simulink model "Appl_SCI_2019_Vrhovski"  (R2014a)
settings: Solver=ode45  StartTime=0.0  StopTime=1000  MaxStep=0.01  RelTol=1e-3
undefined symbols (not defined in the file): deg, H, kg, m, M, mm, N, rad, s, X, Y, Z
libraries: sm_lib x389, nesl_utility x69, simulink x7
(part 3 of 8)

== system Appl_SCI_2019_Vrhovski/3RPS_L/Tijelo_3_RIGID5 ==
  ReferenceFrame : sm_lib/Frames and Transforms/Reference Frame  BlockFunction=simmechanics.library.frames_transforms.reference_frame
  Solid : sm_lib/Body Elements/Solid  InertiaType=Custom  Mass=3.25  MassUnits=kg  CenterOfMass=[0 67.696607712724699 0]  CenterOfMassUnits=mm  MomentsOfInertia=[7450 490 7450]  MomentsOfInertiaUnits=kg*mm^2  ProductsOfInertia=[0 0 0]  ProductsOfInertiaUnits=kg*mm^2  DensityBased=on  Density=1000  DensityUnits=kg/(m^3)  GraphicType=FromGeometry  MarkerShape=Sphere  MarkerSize=10  MarkerSizeUnits=m  GraphicVisPropType=SimpleVisualProperties  GraphicDiffuseColor=[0.4 0.4 0.4]  GraphicSpecularColor=[0.5 0.5 0.5 1.0]  GraphicAmbientColor=[0.15 0.15 0.15 1.0]  GraphicEmissiveColor=[0.0 0.0 0.0 1.0]  GraphicShininess=75  GraphicOpacity=1  GeometryShape=Cylinder  RectangleSize=[1 1]  RectangleSizeUnits=m  BrickDimensions=[1 1 1]  BrickDimensionUnits=m  CylinderRadius=15  CylinderRadiusUnits=mm  CylinderLength=280  CylinderLengthUnits=mm  SphereRadius=1  SphereRadiusUnits=m  EllipsoidRadii=[1 1 1]  EllipsoidRadiiUnits=m  ExtrusionCrossSection=[1 1; -1 1; -1 -1; 1 -1]  ExtrusionCrossSectionUnits=m  ExtrusionLength=1  ExtrusionLengthUnits=m  PolygonNumSides=3  PolygonOuterRadius=1  PolygonOuterRadiusUnits=m  ExtGeomFileType=STL  ExtGeomFileName=Tijelo_Default_sldprt.STL  ExtGeomFileUnits=mm  RevolutionCrossSection=[1 1; 1 -1; 2 -1; 2 1]  RevolutionCrossSectionUnits=m  RevolutionExtent=Full  RevolutionAngle=180  RevolutionAngleUnits=deg  BlockFunction=simmechanics.library.body_elements.solid
  Transform : sm_lib/Frames and Transforms/Rigid Transform  TranslationMethod=StandardAxis  TranslationLengthUnit=mm  TranslationStandardAxis=-Z  TranslationStandardOffset=13.29  TranslationCartesianOffset=[0 10 0]  TranslationROffset=0  TranslationROffsetUnits=m  TranslationZOffset=0  TranslationZOffsetUnits=m  TranslationThetaOffset=0  TranslationThetaOffsetUnits=deg  RotationMethod=None  RotationAngleUnits=rad  RotationStandardAxis=+Z  RotationAngle=2.0943951023931953  RotationArbitraryAxis=[-0.57735026918962584 -0.57735026918962584 -0.57735026918962584]  FollAlignAxisA=+X  BaseAlignAxisA=+Y  FollAlignAxisB=+Y  BaseAlignAxisB=+Z  BlockFunction=simmechanics.library.frames_transforms.rigid_transform
  Transform1 : sm_lib/Frames and Transforms/Rigid Transform  TranslationMethod=None  TranslationLengthUnit=mm  TranslationStandardAxis=+Z  TranslationStandardOffset=0  TranslationCartesianOffset=[0 100 0]  TranslationROffset=0  TranslationROffsetUnits=m  TranslationZOffset=0  TranslationZOffsetUnits=m  TranslationThetaOffset=0  TranslationThetaOffsetUnits=deg  RotationMethod=None  RotationAngleUnits=rad  RotationStandardAxis=+Z  RotationAngle=3.1415926535897905  RotationArbitraryAxis=[1 -1.4003819427637228e-30 -9.8290662577982061e-16]  FollAlignAxisA=+X  BaseAlignAxisA=+Y  FollAlignAxisB=+Y  BaseAlignAxisB=+Z  BlockFunction=simmechanics.library.frames_transforms.rigid_transform
  F1 : PMIOPort  Port=1  Side=Left
  F : PMIOPort  Port=2  Side=Right
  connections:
  Transform1/RConn1 -- F1/RConn1
  Transform/RConn1 -- F/RConn1
  Transform1/LConn1 -- Solid/RConn1 -- ReferenceFrame/RConn1 -- Transform/LConn1

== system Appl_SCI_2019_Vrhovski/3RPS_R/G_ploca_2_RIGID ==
  ReferenceFrame : sm_lib/Frames and Transforms/Reference Frame  BlockFunction=simmechanics.library.frames_transforms.reference_frame
  Solid : sm_lib/Body Elements/Solid  InertiaType=Custom  Mass=5  MassUnits=kg  CenterOfMass=[-1.0925911726464245e-05 0 -4.4436244658035022]  CenterOfMassUnits=mm  MomentsOfInertia=[45540 79860 45540]  MomentsOfInertiaUnits=kg*mm^2  ProductsOfInertia=[0 -0.00010369999054466602 0]  ProductsOfInertiaUnits=kg*mm^2  DensityBased=on  Density=1000  DensityUnits=kg/(m^3)  GraphicType=FromGeometry  MarkerShape=Sphere  MarkerSize=10  MarkerSizeUnits=m  GraphicVisPropType=SimpleVisualProperties  GraphicDiffuseColor=[0.4 0.4 0.4]  GraphicSpecularColor=[0.5 0.5 0.5 1.0]  GraphicAmbientColor=[0.15 0.15 0.15 1.0]  GraphicEmissiveColor=[0.0 0.0 0.0 1.0]  GraphicShininess=75  GraphicOpacity=1  GeometryShape=Brick  RectangleSize=[1 1]  RectangleSizeUnits=m  BrickDimensions=[240 210 20]  BrickDimensionUnits=mm  CylinderRadius=120  CylinderRadiusUnits=mm  CylinderLength=20  CylinderLengthUnits=mm  SphereRadius=1  SphereRadiusUnits=m  EllipsoidRadii=[1 1 1]  EllipsoidRadiiUnits=m  ExtrusionCrossSection=[1 1; -1 1; -1 -1; 1 -1]  ExtrusionCrossSectionUnits=m  ExtrusionLength=1  ExtrusionLengthUnits=m  PolygonNumSides=3  PolygonOuterRadius=1  PolygonOuterRadiusUnits=m  ExtGeomFileType=STL  ExtGeomFileName=G_ploca_Default_sldprt.STL  ExtGeomFileUnits=mm  RevolutionCrossSection=[1 1; 1 -1; 2 -1; 2 1]  RevolutionCrossSectionUnits=m  RevolutionExtent=Full  RevolutionAngle=180  RevolutionAngleUnits=deg  BlockFunction=simmechanics.library.body_elements.solid
  Transform : sm_lib/Frames and Transforms/Rigid Transform  TranslationMethod=Cartesian  TranslationLengthUnit=mm  TranslationStandardAxis=+Z  TranslationStandardOffset=0  TranslationCartesianOffset="[-50.0000   -86.6025         -10]"  TranslationROffset=0  TranslationROffsetUnits=m  TranslationZOffset=0  TranslationZOffsetUnits=m  TranslationThetaOffset=0  TranslationThetaOffsetUnits=deg  RotationMethod=ArbitraryAxis  RotationAngleUnits=rad  RotationStandardAxis=+Z  RotationAngle=0  RotationArbitraryAxis=[0 0 0]  FollAlignAxisA=+X  BaseAlignAxisA=+Y  FollAlignAxisB=+Y  BaseAlignAxisB=+Z  BlockFunction=simmechanics.library.frames_transforms.rigid_transform
  Transform1 : sm_lib/Frames and Transforms/Rigid Transform  TranslationMethod=Cartesian  TranslationLengthUnit=mm  TranslationStandardAxis=+Z  TranslationStandardOffset=0  TranslationCartesianOffset="[-50.0000   86.6025         -10]"  TranslationROffset=0  TranslationROffsetUnits=m  TranslationZOffset=0  TranslationZOffsetUnits=m  TranslationThetaOffset=0  TranslationThetaOffsetUnits=deg  RotationMethod=ArbitraryAxis  RotationAngleUnits=rad  RotationStandardAxis=+Z  RotationAngle=0  RotationArbitraryAxis=[0 0 0]  FollAlignAxisA=+X  BaseAlignAxisA=+Y  FollAlignAxisB=+Y  BaseAlignAxisB=+Z  BlockFunction=simmechanics.library.frames_transforms.rigid_transform
  Transform2 : sm_lib/Frames and Transforms/Rigid Transform  TranslationMethod=Cartesian  TranslationLengthUnit=mm  TranslationStandardAxis=+Z  TranslationStandardOffset=0  TranslationCartesianOffset=[100 0 -10]  TranslationROffset=0  TranslationROffsetUnits=m  TranslationZOffset=0  TranslationZOffsetUnits=m  TranslationThetaOffset=0  TranslationThetaOffsetUnits=deg  RotationMethod=ArbitraryAxis  RotationAngleUnits=rad  RotationStandardAxis=+Z  RotationAngle=0  RotationArbitraryAxis=[0 0 0]  FollAlignAxisA=+X  BaseAlignAxisA=+Y  FollAlignAxisB=+Y  BaseAlignAxisB=+Z  BlockFunction=simmechanics.library.frames_transforms.rigid_transform
  Transform3 : sm_lib/Frames and Transforms/Rigid Transform  TranslationMethod=StandardAxis  TranslationLengthUnit=mm  TranslationStandardAxis=+Z  TranslationStandardOffset=10  TranslationCartesianOffset=[80.000000000002558 4.2632564145606011e-14 -32.999999999999048]  TranslationROffset=0  TranslationROffsetUnits=m  TranslationZOffset=0  TranslationZOffsetUnits=m  TranslationThetaOffset=0  TranslationThetaOffsetUnits=deg  RotationMethod=None  RotationAngleUnits=rad  RotationStandardAxis=+Z  RotationAngle=0  RotationArbitraryAxis=[0 0 0]  FollAlignAxisA=+X  BaseAlignAxisA=+Y  FollAlignAxisB=+Y  BaseAlignAxisB=+Z  BlockFunction=simmechanics.library.frames_transforms.rigid_transform
  F2 : PMIOPort  Port=1  Side=Left
  F1 : PMIOPort  Port=2  Side=Left
  F : PMIOPort  Port=3  Side=Left
  F3 : PMIOPort  Port=4  Side=Right
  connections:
  ReferenceFrame/RConn1 -- Transform/LConn1 -- Transform1/LConn1 -- Transform2/LConn1 -- Transform3/LConn1 -- Solid/RConn1
  Transform/RConn1 -- F/RConn1
  Transform1/RConn1 -- F1/RConn1
  Transform2/RConn1 -- F2/RConn1
  Transform3/RConn1 -- F3/RConn1

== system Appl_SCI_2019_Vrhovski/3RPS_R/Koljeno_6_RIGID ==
  ReferenceFrame : sm_lib/Frames and Transforms/Reference Frame  BlockFunction=simmechanics.library.frames_transforms.reference_frame
  Solid : sm_lib/Body Elements/Solid  InertiaType=Custom  Mass=1.2  MassUnits=kg  CenterOfMass=[0 94.726347166305388 0]  CenterOfMassUnits=mm  MomentsOfInertia=[342 72 342]  MomentsOfInertiaUnits=kg*mm^2  ProductsOfInertia=[0 0 0]  ProductsOfInertiaUnits=kg*mm^2  DensityBased=on  Density=1000  DensityUnits=kg/(m^3)  GraphicType=FromGeometry  MarkerShape=Sphere  MarkerSize=10  MarkerSizeUnits=m  GraphicVisPropType=SimpleVisualProperties  GraphicDiffuseColor=[0.792156862745098 0.81960784313725488 0.93333333333333335]  GraphicSpecularColor=[0.5 0.5 0.5 1.0]  GraphicAmbientColor=[0.15 0.15 0.15 1.0]  GraphicEmissiveColor=[0.0 0.0 0.0 1.0]  GraphicShininess=75  GraphicOpacity=1  GeometryShape=FromFile  RectangleSize=[1 1]  RectangleSizeUnits=m  BrickDimensions=[1 1 1]  BrickDimensionUnits=m  CylinderRadius=1  CylinderRadiusUnits=m  CylinderLength=1  CylinderLengthUnits=m  SphereRadius=1  SphereRadiusUnits=m  EllipsoidRadii=[1 1 1]  EllipsoidRadiiUnits=m  ExtrusionCrossSection=[1 1; -1 1; -1 -1; 1 -1]  ExtrusionCrossSectionUnits=m  ExtrusionLength=1  ExtrusionLengthUnits=m  PolygonNumSides=3  PolygonOuterRadius=1  PolygonOuterRadiusUnits=m  ExtGeomFileType=STL  ExtGeomFileName=E:\Fer 2\Doktorski studij\Doktorat\LLD\matlab\LLD 3RPS\PS_limb.STL  ExtGeomFileUnits=mm  RevolutionCrossSection=[1 1; 1 -1; 2 -1; 2 1]  RevolutionCrossSectionUnits=m  RevolutionExtent=Full  RevolutionAngle=180  RevolutionAngleUnits=deg  BlockFunction=simmechanics.library.body_elements.solid
  Transform : sm_lib/Frames and Transforms/Rigid Transform  TranslationMethod=Cartesian  TranslationLengthUnit=mm  TranslationStandardAxis=+Z  TranslationStandardOffset=0  TranslationCartesianOffset=[2.9560869854197764e-13 -4.9068237247312261e-13 -4.0348858674063459e-14]  TranslationROffset=0  TranslationROffsetUnits=m  TranslationZOffset=0  TranslationZOffsetUnits=m  TranslationThetaOffset=0  TranslationThetaOffsetUnits=deg  RotationMethod=ArbitraryAxis  RotationAngleUnits=rad  RotationStandardAxis=+Z  RotationAngle=2.0943951023931988  RotationArbitraryAxis=[-0.57735026918962673 -0.57735026918962595 -0.57735026918962451]  FollAlignAxisA=+X  BaseAlignAxisA=+Y  FollAlignAxisB=+Y  BaseAlignAxisB=+Z  BlockFunction=simmechanics.library.frames_transforms.rigid_transform
  Transform1 : sm_lib/Frames and Transforms/Rigid Transform  TranslationMethod=Cartesian  TranslationLengthUnit=mm  TranslationStandardAxis=+Z  TranslationStandardOffset=0  TranslationCartesianOffset=[0 162 0]  TranslationROffset=0  TranslationROffsetUnits=m  TranslationZOffset=0  TranslationZOffsetUnits=m  TranslationThetaOffset=0  TranslationThetaOffsetUnits=deg  RotationMethod=ArbitraryAxis  RotationAngleUnits=rad  RotationStandardAxis=+Z  RotationAngle=0  RotationArbitraryAxis=[0 0 0]  FollAlignAxisA=+X  BaseAlignAxisA=+Y  FollAlignAxisB=+Y  BaseAlignAxisB=+Z  BlockFunction=simmechanics.library.frames_transforms.rigid_transform
  F : PMIOPort  Port=1  Side=Left
  F1 : PMIOPort  Port=2  Side=Right
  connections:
  Solid/RConn1 -- ReferenceFrame/RConn1 -- Transform/LConn1 -- Transform1/LConn1
  Transform/RConn1 -- F/RConn1
  Transform1/RConn1 -- F1/RConn1

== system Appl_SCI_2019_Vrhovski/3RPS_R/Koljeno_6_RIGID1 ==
  ReferenceFrame : sm_lib/Frames and Transforms/Reference Frame  BlockFunction=simmechanics.library.frames_transforms.reference_frame
  Solid : sm_lib/Body Elements/Solid  InertiaType=Custom  Mass=1.2  MassUnits=kg  CenterOfMass=[0 94.726347166305388 0]  CenterOfMassUnits=mm  MomentsOfInertia=[342 72 342]  MomentsOfInertiaUnits=kg*mm^2  ProductsOfInertia=[0 0 0]  ProductsOfInertiaUnits=kg*mm^2  DensityBased=on  Density=1000  DensityUnits=kg/(m^3)  GraphicType=FromGeometry  MarkerShape=Sphere  MarkerSize=10  MarkerSizeUnits=m  GraphicVisPropType=SimpleVisualProperties  GraphicDiffuseColor=[0.792156862745098 0.81960784313725488 0.93333333333333335]  GraphicSpecularColor=[0.5 0.5 0.5 1.0]  GraphicAmbientColor=[0.15 0.15 0.15 1.0]  GraphicEmissiveColor=[0.0 0.0 0.0 1.0]  GraphicShininess=75  GraphicOpacity=1  GeometryShape=FromFile  RectangleSize=[1 1]  RectangleSizeUnits=m  BrickDimensions=[1 1 1]  BrickDimensionUnits=m  CylinderRadius=1  CylinderRadiusUnits=m  CylinderLength=1  CylinderLengthUnits=m  SphereRadius=1  SphereRadiusUnits=m  EllipsoidRadii=[1 1 1]  EllipsoidRadiiUnits=m  ExtrusionCrossSection=[1 1; -1 1; -1 -1; 1 -1]  ExtrusionCrossSectionUnits=m  ExtrusionLength=1  ExtrusionLengthUnits=m  PolygonNumSides=3  PolygonOuterRadius=1  PolygonOuterRadiusUnits=m  ExtGeomFileType=STL  ExtGeomFileName=E:\Fer 2\Doktorski studij\Doktorat\LLD\matlab\LLD 3RPS\PS_limb.STL  ExtGeomFileUnits=mm  RevolutionCrossSection=[1 1; 1 -1; 2 -1; 2 1]  RevolutionCrossSectionUnits=m  RevolutionExtent=Full  RevolutionAngle=180  RevolutionAngleUnits=deg  BlockFunction=simmechanics.library.body_elements.solid
  Transform : sm_lib/Frames and Transforms/Rigid Transform  TranslationMethod=Cartesian  TranslationLengthUnit=mm  TranslationStandardAxis=+Z  TranslationStandardOffset=0  TranslationCartesianOffset=[2.9560869854197764e-13 -4.9068237247312261e-13 -4.0348858674063459e-14]  TranslationROffset=0  TranslationROffsetUnits=m  TranslationZOffset=0  TranslationZOffsetUnits=m  TranslationThetaOffset=0  TranslationThetaOffsetUnits=deg  RotationMethod=ArbitraryAxis  RotationAngleUnits=rad  RotationStandardAxis=+Z  RotationAngle=2.0943951023931988  RotationArbitraryAxis=[-0.57735026918962673 -0.57735026918962595 -0.57735026918962451]  FollAlignAxisA=+X  BaseAlignAxisA=+Y  FollAlignAxisB=+Y  BaseAlignAxisB=+Z  BlockFunction=simmechanics.library.frames_transforms.rigid_transform
  Transform1 : sm_lib/Frames and Transforms/Rigid Transform  TranslationMethod=Cartesian  TranslationLengthUnit=mm  TranslationStandardAxis=+Z  TranslationStandardOffset=0  TranslationCartesianOffset=[0 161.99999999999997 0]  TranslationROffset=0  TranslationROffsetUnits=m  TranslationZOffset=0  TranslationZOffsetUnits=m  TranslationThetaOffset=0  TranslationThetaOffsetUnits=deg  RotationMethod=ArbitraryAxis  RotationAngleUnits=rad  RotationStandardAxis=+Z  RotationAngle=0  RotationArbitraryAxis=[0 0 0]  FollAlignAxisA=+X  BaseAlignAxisA=+Y  FollAlignAxisB=+Y  BaseAlignAxisB=+Z  BlockFunction=simmechanics.library.frames_transforms.rigid_transform
  F : PMIOPort  Port=1  Side=Left
  F1 : PMIOPort  Port=2  Side=Right
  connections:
  Transform1/RConn1 -- F1/RConn1
  Transform/RConn1 -- F/RConn1
  Solid/RConn1 -- ReferenceFrame/RConn1 -- Transform1/LConn1 -- Transform/LConn1

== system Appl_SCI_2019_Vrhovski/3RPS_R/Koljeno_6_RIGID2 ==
  ReferenceFrame : sm_lib/Frames and Transforms/Reference Frame  BlockFunction=simmechanics.library.frames_transforms.reference_frame
  Solid : sm_lib/Body Elements/Solid  InertiaType=Custom  Mass=1.2  MassUnits=kg  CenterOfMass=[0 94.726347166305388 0]  CenterOfMassUnits=mm  MomentsOfInertia=[342 72 342]  MomentsOfInertiaUnits=kg*mm^2  ProductsOfInertia=[0 0 0]  ProductsOfInertiaUnits=kg*mm^2  DensityBased=on  Density=1000  DensityUnits=kg/(m^3)  GraphicType=FromGeometry  MarkerShape=Sphere  MarkerSize=10  MarkerSizeUnits=m  GraphicVisPropType=SimpleVisualProperties  GraphicDiffuseColor=[0.792156862745098 0.81960784313725488 0.93333333333333335]  GraphicSpecularColor=[0.5 0.5 0.5 1.0]  GraphicAmbientColor=[0.15 0.15 0.15 1.0]  GraphicEmissiveColor=[0.0 0.0 0.0 1.0]  GraphicShininess=75  GraphicOpacity=1  GeometryShape=FromFile  RectangleSize=[1 1]  RectangleSizeUnits=m  BrickDimensions=[1 1 1]  BrickDimensionUnits=m  CylinderRadius=1  CylinderRadiusUnits=m  CylinderLength=1  CylinderLengthUnits=m  SphereRadius=1  SphereRadiusUnits=m  EllipsoidRadii=[1 1 1]  EllipsoidRadiiUnits=m  ExtrusionCrossSection=[1 1; -1 1; -1 -1; 1 -1]  ExtrusionCrossSectionUnits=m  ExtrusionLength=1  ExtrusionLengthUnits=m  PolygonNumSides=3  PolygonOuterRadius=1  PolygonOuterRadiusUnits=m  ExtGeomFileType=STL  ExtGeomFileName=E:\Fer 2\Doktorski studij\Doktorat\LLD\matlab\LLD 3RPS\PS_limb.STL  ExtGeomFileUnits=mm  RevolutionCrossSection=[1 1; 1 -1; 2 -1; 2 1]  RevolutionCrossSectionUnits=m  RevolutionExtent=Full  RevolutionAngle=180  RevolutionAngleUnits=deg  BlockFunction=simmechanics.library.body_elements.solid
  Transform : sm_lib/Frames and Transforms/Rigid Transform  TranslationMethod=Cartesian  TranslationLengthUnit=mm  TranslationStandardAxis=+Z  TranslationStandardOffset=0  TranslationCartesianOffset=[2.9560869854197764e-13 -4.9068237247312261e-13 -4.0348858674063459e-14]  TranslationROffset=0  TranslationROffsetUnits=m  TranslationZOffset=0  TranslationZOffsetUnits=m  TranslationThetaOffset=0  TranslationThetaOffsetUnits=deg  RotationMethod=ArbitraryAxis  RotationAngleUnits=rad  RotationStandardAxis=+Z  RotationAngle=2.0943951023931988  RotationArbitraryAxis=[-0.57735026918962673 -0.57735026918962595 -0.57735026918962451]  FollAlignAxisA=+X  BaseAlignAxisA=+Y  FollAlignAxisB=+Y  BaseAlignAxisB=+Z  BlockFunction=simmechanics.library.frames_transforms.rigid_transform
  Transform1 : sm_lib/Frames and Transforms/Rigid Transform  TranslationMethod=Cartesian  TranslationLengthUnit=mm  TranslationStandardAxis=+Z  TranslationStandardOffset=0  TranslationCartesianOffset=[0 161.99999999999997 0]  TranslationROffset=0  TranslationROffsetUnits=m  TranslationZOffset=0  TranslationZOffsetUnits=m  TranslationThetaOffset=0  TranslationThetaOffsetUnits=deg  RotationMethod=ArbitraryAxis  RotationAngleUnits=rad  RotationStandardAxis=+Z  RotationAngle=0  RotationArbitraryAxis=[0 0 0]  FollAlignAxisA=+X  BaseAlignAxisA=+Y  FollAlignAxisB=+Y  BaseAlignAxisB=+Z  BlockFunction=simmechanics.library.frames_transforms.rigid_transform
  F : PMIOPort  Port=1  Side=Left
  F1 : PMIOPort  Port=2  Side=Right
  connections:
  Transform/LConn1 -- Transform1/LConn1 -- ReferenceFrame/RConn1 -- Solid/RConn1
  Transform/RConn1 -- F/RConn1
  Transform1/RConn1 -- F1/RConn1

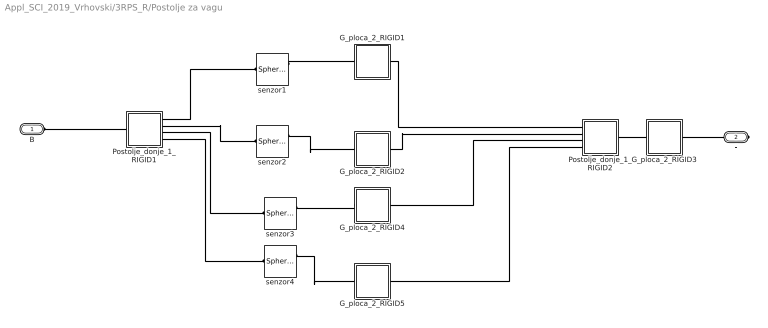
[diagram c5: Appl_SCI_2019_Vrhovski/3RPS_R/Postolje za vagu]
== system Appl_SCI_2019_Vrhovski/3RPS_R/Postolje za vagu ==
  G_ploca_2_RIGID1 : Subsystem
  G_ploca_2_RIGID2 : Subsystem
  G_ploca_2_RIGID3 : Subsystem
  G_ploca_2_RIGID4 : Subsystem
  G_ploca_2_RIGID5 : Subsystem
  Postolje_donje_1_RIGID1 : Subsystem
  Postolje_donje_1_RIGID2 : Subsystem
  senzor{1..4} (4 alike) : sm_lib/Joints/Spherical Joint  SenseConstraintForce=off  SenseConstraintForceX=off  SenseConstraintForceY=off  SenseConstraintForceZ=off  SenseConstraintTorque=off  SenseConstraintTorqueX=off  SenseConstraintTorqueY=off  SenseConstraintTorqueZ=off  SenseTotalForce=on  SenseTotalForceX=off  SenseTotalForceY=off  SenseTotalForceZ=off  SenseTotalTorque=off  SenseTotalTorqueX=off  SenseTotalTorqueY=off  SenseTotalTorqueZ=off  CompositeWrenchDir=FollowerOnBase  CompositeWrenchFrame=BaseFrame  DefPosRotationMethod=None  DefPosRotationAngleUnits=deg  DefPosRotationStandardAxis=+Z  DefPosRotationAngle=0  DefPosRotationArbitraryAxis=[0 0 1]  DefPosFollAlignAxisA=+X  DefPosBaseAlignAxisA=+Y  DefPosFollAlignAxisB=+Y  DefPosBaseAlignAxisB=+Z  EqPosRotationMethod=None  EqPosRotationAngleUnits=deg  EqPosRotationStandardAxis=+Z  EqPosRotationAngle=0  EqPosRotationArbitraryAxis=[0 0 1]  EqPosFollAlignAxisA=+X  EqPosBaseAlignAxisA=+Y  EqPosFollAlignAxisB=+Y  EqPosBaseAlignAxisB=+Z  SpringStiffness=0  SpringStiffnessUnits=m*N/rad  DampingCoefficient=0  DampingCoefficientUnits=m*s*N/rad  ActuateTorqueX=off  ActuateTorqueY=off  ActuateTorqueZ=off  ActuateTorque=off  TorqueActuationMode=NoTorque  MotionActuationMode=ComputedMotion  ActuationFrame=BaseFrame  SensePosition=off  SenseVelocityX=off  SenseVelocityY=off  SenseVelocityZ=off  SenseVelocity=off  SenseAccelerationX=off  SenseAccelerationY=off  SenseAccelerationZ=off  SenseAcceleration=off  SenseTorqueX=off  SenseTorqueY=off  SenseTorqueZ=off  SenseTorqueForce=off  SensingFrame=FollowerFrame  PositionTargetRotationMethod=None  PositionTargetRotationAngleUnits=deg  PositionTargetRotationStandardAxis=+Z  PositionTargetRotationAngle=0  PositionTargetRotationArbitraryAxis=[0 0 1]  PositionTargetFollAlignAxisA=+X  PositionTargetBaseAlignAxisA=+Y  PositionTargetFollAlignAxisB=+Y  PositionTargetBaseAlignAxisB=+Z  PositionTargetSpecify=off  PositionTargetPriority=High  VelocityTargetValue=[0 0 0]  VelocityTargetValueUnits=deg/s  VelocityTargetSpecify=off  VelocityTargetPriority=High  VelocityTargetInFollowerFrame=on  BlockFunction=simmechanics.library.joints.spherical_joint
  B : PMIOPort  Port=1  Side=Left
  F : PMIOPort  Port=2  Side=Right
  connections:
  B/RConn1 -- Postolje_donje_1_RIGID1/LConn1
  G_ploca_2_RIGID4/LConn1 -- senzor3/RConn1
  senzor2/LConn1 -- Postolje_donje_1_RIGID1/RConn2
  senzor4/LConn1 -- Postolje_donje_1_RIGID1/RConn4
  senzor4/RConn1 -- G_ploca_2_RIGID5/LConn1
  G_ploca_2_RIGID1/RConn1 -- Postolje_donje_1_RIGID2/LConn1
  G_ploca_2_RIGID2/RConn1 -- Postolje_donje_1_RIGID2/LConn2
  senzor3/LConn1 -- Postolje_donje_1_RIGID1/RConn3
  G_ploca_2_RIGID5/RConn1 -- Postolje_donje_1_RIGID2/LConn4
  G_ploca_2_RIGID3/RConn1 -- F/RConn1
  G_ploca_2_RIGID3/LConn1 -- Postolje_donje_1_RIGID2/RConn1
  G_ploca_2_RIGID4/RConn1 -- Postolje_donje_1_RIGID2/LConn3
  senzor2/RConn1 -- G_ploca_2_RIGID2/LConn1
  Postolje_donje_1_RIGID1/RConn1 -- senzor1/LConn1
  senzor1/RConn1 -- G_ploca_2_RIGID1/LConn1

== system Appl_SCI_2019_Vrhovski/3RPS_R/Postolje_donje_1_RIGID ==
  ReferenceFrame : sm_lib/Frames and Transforms/Reference Frame  BlockFunction=simmechanics.library.frames_transforms.reference_frame
  Solid : sm_lib/Body Elements/Solid  InertiaType=Custom  Mass=62.206189968539466  MassUnits=kg  CenterOfMass=[0 0 2.5]  CenterOfMassUnits=mm  MomentsOfInertia=[58000.590195722754395 58000.590195722754238 114000.2247851136613]  MomentsOfInertiaUnits=kg*mm^2  ProductsOfInertia=[0 0 0]  ProductsOfInertiaUnits=kg*mm^2  DensityBased=on  Density=10000  DensityUnits=kg/(m^3)  GraphicType=FromGeometry  MarkerShape=Sphere  MarkerSize=10  MarkerSizeUnits=m  GraphicVisPropType=SimpleVisualProperties  GraphicDiffuseColor=[0.4 0.4 0.4]  GraphicSpecularColor=[0.5 0.5 0.5 1.0]  GraphicAmbientColor=[0.15 0.15 0.15 1.0]  GraphicEmissiveColor=[0.0 0.0 0.0 1.0]  GraphicShininess=75  GraphicOpacity=1  GeometryShape=Cylinder  RectangleSize=[1 1]  RectangleSizeUnits=m  BrickDimensions=[300 180 5]  BrickDimensionUnits=mm  CylinderRadius=60  CylinderRadiusUnits=mm  CylinderLength=10  CylinderLengthUnits=mm  SphereRadius=1  SphereRadiusUnits=m  EllipsoidRadii=[1 1 1]  EllipsoidRadiiUnits=m  ExtrusionCrossSection=[1 1; -1 1; -1 -1; 1 -1]  ExtrusionCrossSectionUnits=m  ExtrusionLength=1  ExtrusionLengthUnits=m  PolygonNumSides=3  PolygonOuterRadius=1  PolygonOuterRadiusUnits=m  ExtGeomFileType=STL  ExtGeomFileName=Postolje_donje_Default_sldprt.STL  ExtGeomFileUnits=mm  RevolutionCrossSection=[1 1; 1 -1; 2 -1; 2 1]  RevolutionCrossSectionUnits=m  RevolutionExtent=Full  RevolutionAngle=180  RevolutionAngleUnits=deg  BlockFunction=simmechanics.library.body_elements.solid
  Transform : sm_lib/Frames and Transforms/Rigid Transform  TranslationMethod=Cartesian  TranslationLengthUnit=mm  TranslationStandardAxis=+Z  TranslationStandardOffset=0  TranslationCartesianOffset="[-30.0000   -51.9615         0]"  TranslationROffset=0  TranslationROffsetUnits=m  TranslationZOffset=0  TranslationZOffsetUnits=m  TranslationThetaOffset=0  TranslationThetaOffsetUnits=deg  RotationMethod=ArbitraryAxis  RotationAngleUnits=rad  RotationStandardAxis=+Z  RotationAngle=1.8234765819369776  RotationArbitraryAxis=[0.77459666924148252 0.44721359549995954 0.44721359549995798]  FollAlignAxisA=+X  BaseAlignAxisA=+Y  FollAlignAxisB=+Y  BaseAlignAxisB=+Z  BlockFunction=simmechanics.library.frames_transforms.rigid_transform
  Transform1 : sm_lib/Frames and Transforms/Rigid Transform  TranslationMethod=Cartesian  TranslationLengthUnit=mm  TranslationStandardAxis=+Z  TranslationStandardOffset=0  TranslationCartesianOffset="[ -30.0000   51.9615         0]"  TranslationROffset=0  TranslationROffsetUnits=m  TranslationZOffset=0  TranslationZOffsetUnits=m  TranslationThetaOffset=0  TranslationThetaOffsetUnits=deg  RotationMethod=ArbitraryAxis  RotationAngleUnits=rad  RotationStandardAxis=+Z  RotationAngle=2.41885840577637  RotationArbitraryAxis=[0.37796447300923008 0.65465367070797587 0.65465367070797675]  FollAlignAxisA=+X  BaseAlignAxisA=+Y  FollAlignAxisB=+Y  BaseAlignAxisB=+Z  BlockFunction=simmechanics.library.frames_transforms.rigid_transform
  Transform2 : sm_lib/Frames and Transforms/Rigid Transform  TranslationMethod=Cartesian  TranslationLengthUnit=mm  TranslationStandardAxis=+Z  TranslationStandardOffset=0  TranslationCartesianOffset="[60     0     0]"  TranslationROffset=0  TranslationROffsetUnits=m  TranslationZOffset=0  TranslationZOffsetUnits=m  TranslationThetaOffset=0  TranslationThetaOffsetUnits=deg  RotationMethod=ArbitraryAxis  RotationAngleUnits=rad  RotationStandardAxis=+Z  RotationAngle=2.0943951023931975  RotationArbitraryAxis=[0.57735026918962651 -0.57735026918962651 0.5773502691896244]  FollAlignAxisA=+X  BaseAlignAxisA=+Y  FollAlignAxisB=+Y  BaseAlignAxisB=+Z  BlockFunction=simmechanics.library.frames_transforms.rigid_transform
  F3 : PMIOPort  Port=1  Side=Left
  F2 : PMIOPort  Port=2  Side=Right
  F1 : PMIOPort  Port=3  Side=Right
  F : PMIOPort  Port=4  Side=Right
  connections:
  Transform/RConn1 -- F/RConn1
  Transform1/RConn1 -- F1/RConn1
  Transform2/RConn1 -- F2/RConn1
  Solid/RConn1 -- ReferenceFrame/RConn1 -- Transform2/LConn1 -- Transform1/LConn1 -- Transform/LConn1 -- F3/RConn1

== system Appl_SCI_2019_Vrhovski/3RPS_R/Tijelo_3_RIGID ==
  ReferenceFrame : sm_lib/Frames and Transforms/Reference Frame  BlockFunction=simmechanics.library.frames_transforms.reference_frame
  Solid : sm_lib/Body Elements/Solid  InertiaType=Custom  Mass=3.25  MassUnits=kg  CenterOfMass=[0 67.696607712724699 0]  CenterOfMassUnits=mm  MomentsOfInertia=[7450 490 7450]  MomentsOfInertiaUnits=kg*mm^2  ProductsOfInertia=[0 0 0]  ProductsOfInertiaUnits=kg*mm^2  DensityBased=on  Density=1000  DensityUnits=kg/(m^3)  GraphicType=FromGeometry  MarkerShape=Sphere  MarkerSize=10  MarkerSizeUnits=m  GraphicVisPropType=SimpleVisualProperties  GraphicDiffuseColor=[0.4 0.4 0.4]  GraphicSpecularColor=[0.5 0.5 0.5 1.0]  GraphicAmbientColor=[0.15 0.15 0.15 1.0]  GraphicEmissiveColor=[0.0 0.0 0.0 1.0]  GraphicShininess=75  GraphicOpacity=1  GeometryShape=FromFile  RectangleSize=[1 1]  RectangleSizeUnits=m  BrickDimensions=[1 1 1]  BrickDimensionUnits=m  CylinderRadius=1  CylinderRadiusUnits=m  CylinderLength=1  CylinderLengthUnits=m  SphereRadius=1  SphereRadiusUnits=m  EllipsoidRadii=[1 1 1]  EllipsoidRadiiUnits=m  ExtrusionCrossSection=[1 1; -1 1; -1 -1; 1 -1]  ExtrusionCrossSectionUnits=m  ExtrusionLength=1  ExtrusionLengthUnits=m  PolygonNumSides=3  PolygonOuterRadius=1  PolygonOuterRadiusUnits=m  ExtGeomFileType=STL  ExtGeomFileName=E:\Fer 2\Doktorski studij\Doktorat\LLD\matlab\LLD 3RPS\RP_limb.STL  ExtGeomFileUnits=mm  RevolutionCrossSection=[1 1; 1 -1; 2 -1; 2 1]  RevolutionCrossSectionUnits=m  RevolutionExtent=Full  RevolutionAngle=180  RevolutionAngleUnits=deg  BlockFunction=simmechanics.library.body_elements.solid
  Transform : sm_lib/Frames and Transforms/Rigid Transform  TranslationMethod=Cartesian  TranslationLengthUnit=mm  TranslationStandardAxis=+Z  TranslationStandardOffset=0  TranslationCartesianOffset=[0 150 0]  TranslationROffset=0  TranslationROffsetUnits=m  TranslationZOffset=0  TranslationZOffsetUnits=m  TranslationThetaOffset=0  TranslationThetaOffsetUnits=deg  RotationMethod=ArbitraryAxis  RotationAngleUnits=rad  RotationStandardAxis=+Z  RotationAngle=2.0943951023931953  RotationArbitraryAxis=[-0.57735026918962584 -0.57735026918962584 -0.57735026918962584]  FollAlignAxisA=+X  BaseAlignAxisA=+Y  FollAlignAxisB=+Y  BaseAlignAxisB=+Z  BlockFunction=simmechanics.library.frames_transforms.rigid_transform
  Transform1 : sm_lib/Frames and Transforms/Rigid Transform  TranslationMethod=Cartesian  TranslationLengthUnit=mm  TranslationStandardAxis=+Z  TranslationStandardOffset=0  TranslationCartesianOffset=[0 -10 0]  TranslationROffset=0  TranslationROffsetUnits=m  TranslationZOffset=0  TranslationZOffsetUnits=m  TranslationThetaOffset=0  TranslationThetaOffsetUnits=deg  RotationMethod=ArbitraryAxis  RotationAngleUnits=rad  RotationStandardAxis=+Z  RotationAngle=3.1415926535897905  RotationArbitraryAxis=[1 -1.4003819427637228e-30 -9.8290662577982061e-16]  FollAlignAxisA=+X  BaseAlignAxisA=+Y  FollAlignAxisB=+Y  BaseAlignAxisB=+Z  BlockFunction=simmechanics.library.frames_transforms.rigid_transform
  F1 : PMIOPort  Port=1  Side=Left
  F : PMIOPort  Port=2  Side=Right
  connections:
  Solid/RConn1 -- ReferenceFrame/RConn1 -- Transform/LConn1 -- Transform1/LConn1
  Transform/RConn1 -- F/RConn1
  Transform1/RConn1 -- F1/RConn1

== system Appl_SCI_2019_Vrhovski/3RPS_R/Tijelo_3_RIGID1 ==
  ReferenceFrame : sm_lib/Frames and Transforms/Reference Frame  BlockFunction=simmechanics.library.frames_transforms.reference_frame
  Solid : sm_lib/Body Elements/Solid  InertiaType=Custom  Mass=3.25  MassUnits=kg  CenterOfMass=[0 67.696607712724699 0]  CenterOfMassUnits=mm  MomentsOfInertia=[7450 490 7450]  MomentsOfInertiaUnits=kg*mm^2  ProductsOfInertia=[0 0 0]  ProductsOfInertiaUnits=kg*mm^2  DensityBased=on  Density=1000  DensityUnits=kg/(m^3)  GraphicType=FromGeometry  MarkerShape=Sphere  MarkerSize=10  MarkerSizeUnits=m  GraphicVisPropType=SimpleVisualProperties  GraphicDiffuseColor=[0.4 0.4 0.4]  GraphicSpecularColor=[0.5 0.5 0.5 1.0]  GraphicAmbientColor=[0.15 0.15 0.15 1.0]  GraphicEmissiveColor=[0.0 0.0 0.0 1.0]  GraphicShininess=75  GraphicOpacity=1  GeometryShape=FromFile  RectangleSize=[1 1]  RectangleSizeUnits=m  BrickDimensions=[1 1 1]  BrickDimensionUnits=m  CylinderRadius=1  CylinderRadiusUnits=m  CylinderLength=1  CylinderLengthUnits=m  SphereRadius=1  SphereRadiusUnits=m  EllipsoidRadii=[1 1 1]  EllipsoidRadiiUnits=m  ExtrusionCrossSection=[1 1; -1 1; -1 -1; 1 -1]  ExtrusionCrossSectionUnits=m  ExtrusionLength=1  ExtrusionLengthUnits=m  PolygonNumSides=3  PolygonOuterRadius=1  PolygonOuterRadiusUnits=m  ExtGeomFileType=STL  ExtGeomFileName=E:\Fer 2\Doktorski studij\Doktorat\LLD\matlab\LLD 3RPS\RP_limb.STL  ExtGeomFileUnits=mm  RevolutionCrossSection=[1 1; 1 -1; 2 -1; 2 1]  RevolutionCrossSectionUnits=m  RevolutionExtent=Full  RevolutionAngle=180  RevolutionAngleUnits=deg  BlockFunction=simmechanics.library.body_elements.solid
  Transform : sm_lib/Frames and Transforms/Rigid Transform  TranslationMethod=Cartesian  TranslationLengthUnit=mm  TranslationStandardAxis=+Z  TranslationStandardOffset=0  TranslationCartesianOffset=[0 150 0]  TranslationROffset=0  TranslationROffsetUnits=m  TranslationZOffset=0  TranslationZOffsetUnits=m  TranslationThetaOffset=0  TranslationThetaOffsetUnits=deg  RotationMethod=ArbitraryAxis  RotationAngleUnits=rad  RotationStandardAxis=+Z  RotationAngle=2.0943951023931953  RotationArbitraryAxis=[-0.57735026918962584 -0.57735026918962584 -0.57735026918962584]  FollAlignAxisA=+X  BaseAlignAxisA=+Y  FollAlignAxisB=+Y  BaseAlignAxisB=+Z  BlockFunction=simmechanics.library.frames_transforms.rigid_transform
  Transform1 : sm_lib/Frames and Transforms/Rigid Transform  TranslationMethod=Cartesian  TranslationLengthUnit=mm  TranslationStandardAxis=+Z  TranslationStandardOffset=0  TranslationCartesianOffset=[0 -10 0]  TranslationROffset=0  TranslationROffsetUnits=m  TranslationZOffset=0  TranslationZOffsetUnits=m  TranslationThetaOffset=0  TranslationThetaOffsetUnits=deg  RotationMethod=ArbitraryAxis  RotationAngleUnits=rad  RotationStandardAxis=+Z  RotationAngle=3.1415926535897905  RotationArbitraryAxis=[1 -1.4003819427637228e-30 -9.8290662577982061e-16]  FollAlignAxisA=+X  BaseAlignAxisA=+Y  FollAlignAxisB=+Y  BaseAlignAxisB=+Z  BlockFunction=simmechanics.library.frames_transforms.rigid_transform
  F1 : PMIOPort  Port=1  Side=Left
  F : PMIOPort  Port=2  Side=Right
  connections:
  Transform1/RConn1 -- F1/RConn1
  Transform/RConn1 -- F/RConn1
  ReferenceFrame/RConn1 -- Solid/RConn1 -- Transform1/LConn1 -- Transform/LConn1

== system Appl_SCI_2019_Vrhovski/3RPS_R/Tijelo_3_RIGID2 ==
  ReferenceFrame : sm_lib/Frames and Transforms/Reference Frame  BlockFunction=simmechanics.library.frames_transforms.reference_frame
  Solid : sm_lib/Body Elements/Solid  InertiaType=Custom  Mass=3.25  MassUnits=kg  CenterOfMass=[0 67.696607712724699 0]  CenterOfMassUnits=mm  MomentsOfInertia=[7450 490 7450]  MomentsOfInertiaUnits=kg*mm^2  ProductsOfInertia=[0 0 0]  ProductsOfInertiaUnits=kg*mm^2  DensityBased=on  Density=1000  DensityUnits=kg/(m^3)  GraphicType=FromGeometry  MarkerShape=Sphere  MarkerSize=10  MarkerSizeUnits=m  GraphicVisPropType=SimpleVisualProperties  GraphicDiffuseColor=[0.4 0.4 0.4]  GraphicSpecularColor=[0.5 0.5 0.5 1.0]  GraphicAmbientColor=[0.15 0.15 0.15 1.0]  GraphicEmissiveColor=[0.0 0.0 0.0 1.0]  GraphicShininess=75  GraphicOpacity=1  GeometryShape=FromFile  RectangleSize=[1 1]  RectangleSizeUnits=m  BrickDimensions=[1 1 1]  BrickDimensionUnits=m  CylinderRadius=1  CylinderRadiusUnits=m  CylinderLength=1  CylinderLengthUnits=m  SphereRadius=1  SphereRadiusUnits=m  EllipsoidRadii=[1 1 1]  EllipsoidRadiiUnits=m  ExtrusionCrossSection=[1 1; -1 1; -1 -1; 1 -1]  ExtrusionCrossSectionUnits=m  ExtrusionLength=1  ExtrusionLengthUnits=m  PolygonNumSides=3  PolygonOuterRadius=1  PolygonOuterRadiusUnits=m  ExtGeomFileType=STL  ExtGeomFileName=E:\Fer 2\Doktorski studij\Doktorat\LLD\matlab\LLD 3RPS\RP_limb.STL  ExtGeomFileUnits=mm  RevolutionCrossSection=[1 1; 1 -1; 2 -1; 2 1]  RevolutionCrossSectionUnits=m  RevolutionExtent=Full  RevolutionAngle=180  RevolutionAngleUnits=deg  BlockFunction=simmechanics.library.body_elements.solid
  Transform : sm_lib/Frames and Transforms/Rigid Transform  TranslationMethod=Cartesian  TranslationLengthUnit=mm  TranslationStandardAxis=+Z  TranslationStandardOffset=0  TranslationCartesianOffset=[0 150 0]  TranslationROffset=0  TranslationROffsetUnits=m  TranslationZOffset=0  TranslationZOffsetUnits=m  TranslationThetaOffset=0  TranslationThetaOffsetUnits=deg  RotationMethod=ArbitraryAxis  RotationAngleUnits=rad  RotationStandardAxis=+Z  RotationAngle=2.0943951023931953  RotationArbitraryAxis=[-0.57735026918962584 -0.57735026918962584 -0.57735026918962584]  FollAlignAxisA=+X  BaseAlignAxisA=+Y  FollAlignAxisB=+Y  BaseAlignAxisB=+Z  BlockFunction=simmechanics.library.frames_transforms.rigid_transform
  Transform1 : sm_lib/Frames and Transforms/Rigid Transform  TranslationMethod=Cartesian  TranslationLengthUnit=mm  TranslationStandardAxis=+Z  TranslationStandardOffset=0  TranslationCartesianOffset=[0 -10 0]  TranslationROffset=0  TranslationROffsetUnits=m  TranslationZOffset=0  TranslationZOffsetUnits=m  TranslationThetaOffset=0  TranslationThetaOffsetUnits=deg  RotationMethod=ArbitraryAxis  RotationAngleUnits=rad  RotationStandardAxis=+Z  RotationAngle=3.1415926535897905  RotationArbitraryAxis=[1 -1.4003819427637228e-30 -9.8290662577982061e-16]  FollAlignAxisA=+X  BaseAlignAxisA=+Y  FollAlignAxisB=+Y  BaseAlignAxisB=+Z  BlockFunction=simmechanics.library.frames_transforms.rigid_transform
  F1 : PMIOPort  Port=1  Side=Left
  F : PMIOPort  Port=2  Side=Right
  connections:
  Transform/LConn1 -- Transform1/LConn1 -- Solid/RConn1 -- ReferenceFrame/RConn1
  Transform/RConn1 -- F/RConn1
  Transform1/RConn1 -- F1/RConn1

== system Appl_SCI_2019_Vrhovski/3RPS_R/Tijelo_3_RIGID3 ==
  ReferenceFrame : sm_lib/Frames and Transforms/Reference Frame  BlockFunction=simmechanics.library.frames_transforms.reference_frame
  Solid : sm_lib/Body Elements/Solid  InertiaType=Custom  Mass=3.25  MassUnits=kg  CenterOfMass=[0 67.696607712724699 0]  CenterOfMassUnits=mm  MomentsOfInertia=[7450 490 7450]  MomentsOfInertiaUnits=kg*mm^2  ProductsOfInertia=[0 0 0]  ProductsOfInertiaUnits=kg*mm^2  DensityBased=on  Density=1000  DensityUnits=kg/(m^3)  GraphicType=FromGeometry  MarkerShape=Sphere  MarkerSize=10  MarkerSizeUnits=m  GraphicVisPropType=SimpleVisualProperties  GraphicDiffuseColor=[0.4 0.4 0.4]  GraphicSpecularColor=[0.5 0.5 0.5 1.0]  GraphicAmbientColor=[0.15 0.15 0.15 1.0]  GraphicEmissiveColor=[0.0 0.0 0.0 1.0]  GraphicShininess=75  GraphicOpacity=1  GeometryShape=Cylinder  RectangleSize=[1 1]  RectangleSizeUnits=m  BrickDimensions=[1 1 1]  BrickDimensionUnits=m  CylinderRadius=15  CylinderRadiusUnits=mm  CylinderLength=280  CylinderLengthUnits=mm  SphereRadius=1  SphereRadiusUnits=m  EllipsoidRadii=[1 1 1]  EllipsoidRadiiUnits=m  ExtrusionCrossSection=[1 1; -1 1; -1 -1; 1 -1]  ExtrusionCrossSectionUnits=m  ExtrusionLength=1  ExtrusionLengthUnits=m  PolygonNumSides=3  PolygonOuterRadius=1  PolygonOuterRadiusUnits=m  ExtGeomFileType=STL  ExtGeomFileName=Tijelo_Default_sldprt.STL  ExtGeomFileUnits=mm  RevolutionCrossSection=[1 1; 1 -1; 2 -1; 2 1]  RevolutionCrossSectionUnits=m  RevolutionExtent=Full  RevolutionAngle=180  RevolutionAngleUnits=deg  BlockFunction=simmechanics.library.body_elements.solid
  Transform : sm_lib/Frames and Transforms/Rigid Transform  TranslationMethod=StandardAxis  TranslationLengthUnit=mm  TranslationStandardAxis=-Z  TranslationStandardOffset=13.29  TranslationCartesianOffset=[0 10 0]  TranslationROffset=0  TranslationROffsetUnits=m  TranslationZOffset=0  TranslationZOffsetUnits=m  TranslationThetaOffset=0  TranslationThetaOffsetUnits=deg  RotationMethod=None  RotationAngleUnits=rad  RotationStandardAxis=+Z  RotationAngle=2.0943951023931953  RotationArbitraryAxis=[-0.57735026918962584 -0.57735026918962584 -0.57735026918962584]  FollAlignAxisA=+X  BaseAlignAxisA=+Y  FollAlignAxisB=+Y  BaseAlignAxisB=+Z  BlockFunction=simmechanics.library.frames_transforms.rigid_transform
  Transform1 : sm_lib/Frames and Transforms/Rigid Transform  TranslationMethod=None  TranslationLengthUnit=mm  TranslationStandardAxis=+Z  TranslationStandardOffset=0  TranslationCartesianOffset=[0 100 0]  TranslationROffset=0  TranslationROffsetUnits=m  TranslationZOffset=0  TranslationZOffsetUnits=m  TranslationThetaOffset=0  TranslationThetaOffsetUnits=deg  RotationMethod=None  RotationAngleUnits=rad  RotationStandardAxis=+Z  RotationAngle=3.1415926535897905  RotationArbitraryAxis=[1 -1.4003819427637228e-30 -9.8290662577982061e-16]  FollAlignAxisA=+X  BaseAlignAxisA=+Y  FollAlignAxisB=+Y  BaseAlignAxisB=+Z  BlockFunction=simmechanics.library.frames_transforms.rigid_transform
  F1 : PMIOPort  Port=1  Side=Left
  F : PMIOPort  Port=2  Side=Right
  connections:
  Transform1/RConn1 -- F1/RConn1
  Transform/RConn1 -- F/RConn1
  Transform1/LConn1 -- Transform/LConn1 -- ReferenceFrame/RConn1 -- Solid/RConn1

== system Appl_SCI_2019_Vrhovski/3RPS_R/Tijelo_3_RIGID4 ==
  ReferenceFrame : sm_lib/Frames and Transforms/Reference Frame  BlockFunction=simmechanics.library.frames_transforms.reference_frame
  Solid : sm_lib/Body Elements/Solid  InertiaType=Custom  Mass=3.25  MassUnits=kg  CenterOfMass=[0 67.696607712724699 0]  CenterOfMassUnits=mm  MomentsOfInertia=[7450 490 7450]  MomentsOfInertiaUnits=kg*mm^2  ProductsOfInertia=[0 0 0]  ProductsOfInertiaUnits=kg*mm^2  DensityBased=on  Density=1000  DensityUnits=kg/(m^3)  GraphicType=FromGeometry  MarkerShape=Sphere  MarkerSize=10  MarkerSizeUnits=m  GraphicVisPropType=SimpleVisualProperties  GraphicDiffuseColor=[0.4 0.4 0.4]  GraphicSpecularColor=[0.5 0.5 0.5 1.0]  GraphicAmbientColor=[0.15 0.15 0.15 1.0]  GraphicEmissiveColor=[0.0 0.0 0.0 1.0]  GraphicShininess=75  GraphicOpacity=1  GeometryShape=Cylinder  RectangleSize=[1 1]  RectangleSizeUnits=m  BrickDimensions=[1 1 1]  BrickDimensionUnits=m  CylinderRadius=15  CylinderRadiusUnits=mm  CylinderLength=280  CylinderLengthUnits=mm  SphereRadius=1  SphereRadiusUnits=m  EllipsoidRadii=[1 1 1]  EllipsoidRadiiUnits=m  ExtrusionCrossSection=[1 1; -1 1; -1 -1; 1 -1]  ExtrusionCrossSectionUnits=m  ExtrusionLength=1  ExtrusionLengthUnits=m  PolygonNumSides=3  PolygonOuterRadius=1  PolygonOuterRadiusUnits=m  ExtGeomFileType=STL  ExtGeomFileName=Tijelo_Default_sldprt.STL  ExtGeomFileUnits=mm  RevolutionCrossSection=[1 1; 1 -1; 2 -1; 2 1]  RevolutionCrossSectionUnits=m  RevolutionExtent=Full  RevolutionAngle=180  RevolutionAngleUnits=deg  BlockFunction=simmechanics.library.body_elements.solid
  Transform : sm_lib/Frames and Transforms/Rigid Transform  TranslationMethod=StandardAxis  TranslationLengthUnit=mm  TranslationStandardAxis=-Z  TranslationStandardOffset=13.29  TranslationCartesianOffset=[0 10 0]  TranslationROffset=0  TranslationROffsetUnits=m  TranslationZOffset=0  TranslationZOffsetUnits=m  TranslationThetaOffset=0  TranslationThetaOffsetUnits=deg  RotationMethod=None  RotationAngleUnits=rad  RotationStandardAxis=+Z  RotationAngle=2.0943951023931953  RotationArbitraryAxis=[-0.57735026918962584 -0.57735026918962584 -0.57735026918962584]  FollAlignAxisA=+X  BaseAlignAxisA=+Y  FollAlignAxisB=+Y  BaseAlignAxisB=+Z  BlockFunction=simmechanics.library.frames_transforms.rigid_transform
  Transform1 : sm_lib/Frames and Transforms/Rigid Transform  TranslationMethod=None  TranslationLengthUnit=mm  TranslationStandardAxis=+Z  TranslationStandardOffset=0  TranslationCartesianOffset=[0 100 0]  TranslationROffset=0  TranslationROffsetUnits=m  TranslationZOffset=0  TranslationZOffsetUnits=m  TranslationThetaOffset=0  TranslationThetaOffsetUnits=deg  RotationMethod=None  RotationAngleUnits=rad  RotationStandardAxis=+Z  RotationAngle=3.1415926535897905  RotationArbitraryAxis=[1 -1.4003819427637228e-30 -9.8290662577982061e-16]  FollAlignAxisA=+X  BaseAlignAxisA=+Y  FollAlignAxisB=+Y  BaseAlignAxisB=+Z  BlockFunction=simmechanics.library.frames_transforms.rigid_transform
  F1 : PMIOPort  Port=1  Side=Left
  F : PMIOPort  Port=2  Side=Right
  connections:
  ReferenceFrame/RConn1 -- Solid/RConn1 -- Transform1/LConn1 -- Transform/LConn1
  Transform/RConn1 -- F/RConn1
  Transform1/RConn1 -- F1/RConn1

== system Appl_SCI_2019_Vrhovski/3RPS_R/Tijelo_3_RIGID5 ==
  ReferenceFrame : sm_lib/Frames and Transforms/Reference Frame  BlockFunction=simmechanics.library.frames_transforms.reference_frame
  Solid : sm_lib/Body Elements/Solid  InertiaType=Custom  Mass=3.25  MassUnits=kg  CenterOfMass=[0 67.696607712724699 0]  CenterOfMassUnits=mm  MomentsOfInertia=[7450 490 7450]  MomentsOfInertiaUnits=kg*mm^2  ProductsOfInertia=[0 0 0]  ProductsOfInertiaUnits=kg*mm^2  DensityBased=on  Density=1000  DensityUnits=kg/(m^3)  GraphicType=FromGeometry  MarkerShape=Sphere  MarkerSize=10  MarkerSizeUnits=m  GraphicVisPropType=SimpleVisualProperties  GraphicDiffuseColor=[0.4 0.4 0.4]  GraphicSpecularColor=[0.5 0.5 0.5 1.0]  GraphicAmbientColor=[0.15 0.15 0.15 1.0]  GraphicEmissiveColor=[0.0 0.0 0.0 1.0]  GraphicShininess=75  GraphicOpacity=1  GeometryShape=Cylinder  RectangleSize=[1 1]  RectangleSizeUnits=m  BrickDimensions=[1 1 1]  BrickDimensionUnits=m  CylinderRadius=15  CylinderRadiusUnits=mm  CylinderLength=280  CylinderLengthUnits=mm  SphereRadius=1  SphereRadiusUnits=m  EllipsoidRadii=[1 1 1]  EllipsoidRadiiUnits=m  ExtrusionCrossSection=[1 1; -1 1; -1 -1; 1 -1]  ExtrusionCrossSectionUnits=m  ExtrusionLength=1  ExtrusionLengthUnits=m  PolygonNumSides=3  PolygonOuterRadius=1  PolygonOuterRadiusUnits=m  ExtGeomFileType=STL  ExtGeomFileName=Tijelo_Default_sldprt.STL  ExtGeomFileUnits=mm  RevolutionCrossSection=[1 1; 1 -1; 2 -1; 2 1]  RevolutionCrossSectionUnits=m  RevolutionExtent=Full  RevolutionAngle=180  RevolutionAngleUnits=deg  BlockFunction=simmechanics.library.body_elements.solid
  Transform : sm_lib/Frames and Transforms/Rigid Transform  TranslationMethod=StandardAxis  TranslationLengthUnit=mm  TranslationStandardAxis=-Z  TranslationStandardOffset=13.29  TranslationCartesianOffset=[0 10 0]  TranslationROffset=0  TranslationROffsetUnits=m  TranslationZOffset=0  TranslationZOffsetUnits=m  TranslationThetaOffset=0  TranslationThetaOffsetUnits=deg  RotationMethod=None  RotationAngleUnits=rad  RotationStandardAxis=+Z  RotationAngle=2.0943951023931953  RotationArbitraryAxis=[-0.57735026918962584 -0.57735026918962584 -0.57735026918962584]  FollAlignAxisA=+X  BaseAlignAxisA=+Y  FollAlignAxisB=+Y  BaseAlignAxisB=+Z  BlockFunction=simmechanics.library.frames_transforms.rigid_transform
  Transform1 : sm_lib/Frames and Transforms/Rigid Transform  TranslationMethod=None  TranslationLengthUnit=mm  TranslationStandardAxis=+Z  TranslationStandardOffset=0  TranslationCartesianOffset=[0 100 0]  TranslationROffset=0  TranslationROffsetUnits=m  TranslationZOffset=0  TranslationZOffsetUnits=m  TranslationThetaOffset=0  TranslationThetaOffsetUnits=deg  RotationMethod=None  RotationAngleUnits=rad  RotationStandardAxis=+Z  RotationAngle=3.1415926535897905  RotationArbitraryAxis=[1 -1.4003819427637228e-30 -9.8290662577982061e-16]  FollAlignAxisA=+X  BaseAlignAxisA=+Y  FollAlignAxisB=+Y  BaseAlignAxisB=+Z  BlockFunction=simmechanics.library.frames_transforms.rigid_transform
  F1 : PMIOPort  Port=1  Side=Left
  F : PMIOPort  Port=2  Side=Right
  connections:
  Transform1/RConn1 -- F1/RConn1
  Transform/RConn1 -- F/RConn1
  Transform1/LConn1 -- Solid/RConn1 -- ReferenceFrame/RConn1 -- Transform/LConn1
